| IBIS file p1010_ibis.ibs generated by Viper version: 2010.05.25
[IBIS Ver]   4.2
[Comment Char]   |_char
[File Name]   p1010_ibis.ibs
[File Rev]   E
[Date]   Mon Feb 18 04:38:39 2013
[Source]
[Notes]   Added models for ddr3 Full & Half strength .
|File Rev A : It is generated with the existing lvcmos & ddr models.
|File Rev B : It is updated with insertion of ddr3 Full & Half strength ddr3 models.
|FIle Rev C : It is further updated with the ddr3 /ddr3l input models with ODT Values for full stregth & Half Strength.
|FIle Rev D : Updated Vinl and Vinh value for ddr3 /ddr3l
|FIle Rev E : Expanded Vin data  for ddr3 /ddr3l
|DDR3/DDR3L Input models with ODT for full strength
|v135_in_wb_fs20_term_40_111
|v135_in_wb_fs20_term_45_110
|v135_in_wb_fs20_term_50_101
|v135_in_wb_fs20_term_50_100
|v135_in_wb_fs20_term_100_011
|v135_in_wb_fs20_noterm_000
|v150_in_wb_fs20_term_40_111
|v150_in_wb_fs20_term_45_110
|v150_in_wb_fs20_term_50_101
|v150_in_wb_fs20_term_60_010
|v150_in_wb_fs20_term_150_001
|v150_in_wb_fs20_noterm_000
|DDR3/DDR3L Input models with ODT for default/Half strength
|v135_in_wb_term_40_111
|v135_in_wb_term_45_110
|v135_in_wb_term_50_101
|v135_in_wb_term_50_100
|v135_in_wb_term_100_011
|v135_in_wb_noterm_000
|v150_in_wb_term_40_111
|v150_in_wb_term_45_110
|v150_in_wb_term_50_101
|v150_in_wb_term_60_010
|v150_in_wb_term_150_001
|v150_in_wb_noterm_000
|V135 corresponds to 1.35 volt ddr3l ibis model
|V150 corresponds to 1.50 volt ddr3 ibis model
[Disclaimer] IMPORTANT NOTICE
  This information is provided on an AS IS basis and without warranty.
  IN NO EVENT SHALL Freescale BE LIABLE FOR INCIDENTAL OR CONSEQUENTIAL
  DAMAGES ARISING FROM USE OF THIS INFORMATION. THIS DISCLAIMER OF
  WARRANTY EXTENDS TO THE USER OF THE INFORMATION, AND TO THEIR CUSTOMERS
  OR USERS OF PRODUCTS  AND IS IN LIEU OF ALL WARRANTIES WHETHER EXPRESS,
  IMPLIED, OR STATUTORY, INCLUDING IMPLIED WARRANTIES OF MERCHANTABILITY
  OR FITNESS FOR PARTICULAR PURPOSE.
  Freescale does not represent or warrant that the information furnished
  hereunder is free of infringement of any third party patents,
  copyrights, trade secrets, or other intellectual property rights.
  Freescale does not represent or warrant that the information is free of
  defect, or that it meets any particular standard, requirements or need
  of the user of the infomation or their customers.
  Freescale reserves the right to change the information in this file
  without notice.
[Copyright]   (C) Copyright Freescale 2004 - 2010, All Rights Reserved.
|   P1010
[Component]   P1010
[Manufacturer]   FREESCALE
[Package]
| variable   typ   min   max
R_pkg   0.5638290   0.004778   0.709444
L_pkg   4.99081nH   0.08270nH   8.13625nH
C_pkg   1.95489pF   0.77573pF   61.6917pF
[Pin] signal_name   model_name   R_pin   L_pin   C_pin
A1   VSS   GND   NA   NA   NA
A2   MA4   ddr3_lp   0.669707  7.47435nH 1.33505pF
A3   MA7   ddr3_lp   0.637736  6.2879nH  1.1992pF
A4   MA11   ddr3_lp   0.632318  6.08385nH 1.06391pF
A5   MA6   ddr3_lp   0.616007  5.85776nH 1.13647pF
A6   MA13   ddr3_lp   0.647612  6.15309nH 0.92985pF
A7   MA15   ddr3_lp   0.639758  6.02845nH 0.99263pF
A8   MCS2_B   ddr3_lp   0.588837  6.64056nH 0.93350pF
A9   VSS   GND   NA   NA   NA
A10   S2VDD   POWER   0.0536342 0.77289nH 10.8238pF
A11   SD2_RXE_P   ptrmr100_cm   0.617825  4.91248nH 1.00415pF
A12   S2VDD   POWER   0.0536342 0.77289nH 10.8238pF
A13   SD2_RXA_P   ptrmr100_cm   0.651909  5.19846nH 0.88242pF
A14   X2VDD   POWER   0.0841892 1.09167nH 7.24723pF
A15   VSS   GND   NA   NA   NA
A16   SPI_MOSI   lvcmos   0.625378  6.00035nH 1.0182pF
A17   CAN1_TX   lvcmos   0.611521  5.40587nH 1.08898pF
A18   CAN2_TX   lvcmos   0.638959  6.18092nH 1.00055pF
A19   UART_CTS_B00   lvcmos   0.638349  5.85583nH 0.93401pF
A20   UART_CTS_B01   lvcmos   0.662822  6.52645nH 0.90542pF
A21   IIC1_SDA   lvcmos   0.693375  6.89901nH 1.03172pF
A22   IIC2_SDA   lvcmos   0.690978  6.7034nH  1.2023pF
A23   GPIO02   lvcmos   0.670586  6.92508nH 1.28436pF
B1   MCS0_B   ddr3_lp   0.633996  6.98587nH 1.34917pF
B3   MA3   ddr3_lp   0.673586  6.26512nH 1.29594pF
B4   VSS   GND   NA   NA   NA
B5   MA9   ddr3_lp   0.647296  5.55788nH 1.12941pF
B6   MA2   ddr3_lp   0.628027  5.34605nH 1.05351pF
B7   VSS   GND   NA   NA   NA
B8   MCS3_B   ddr3_lp   0.627363  6.05786nH 0.91183pF
B9   X2VDD   POWER   0.0841892 1.09167nH 7.24723pF
B10   S2VSS   GND   NA   NA   NA
B11   SD2_RXE_N   ptrmr100_cm   0.619546  4.93621nH 1.04449pF
B12   S2VSS   GND   NA   NA   NA
B13   SD2_RXA_N   ptrmr100_cm   0.641883  5.19633nH 0.86855pF
B14   X2VSS   GND   NA   NA   NA
B15   X2VSS   GND   NA   NA   NA
B16   SPI_MISO   lvcmos   0.576792  5.7496nH  1.05876pF
B17   VSS   GND   NA   NA   NA
B18   CAN2_RX   lvcmos   0.561266  4.84225nH 1.13305pF
B19   VSS   GND   NA   NA   NA
B20   IIC1_SCL   lvcmos   0.619918  5.55105nH 1.20145pF
B21   GPIO04   lvcmos   0.667179  6.19423nH 1.30918pF
B22   VSS   GND   NA   NA   NA
B23   GPIO03   lvcmos   0.599915  6.11729nH 1.26323pF
C1   MCKE1   ddr3_lp   0.610929  6.46005nH 1.3986pF
C2   MCS1_B   ddr3_lp   0.566315  6.21152nH 1.28084pF
C3   MA14   ddr3_lp   0.666391  6.00916nH 1.29268pF
C4   MBA0   ddr3_lp   0.601323  5.2337nH  1.2176pF
C5   MBA1   ddr3_lp   0.628619  5.18829nH 1.03111pF
C6   MA8   ddr3_lp   0.595826  5.24786nH 1.32086pF
C7   MA5   ddr3_lp   0.58023   5.04038nH 1.11881pF
C8   MDIC1   ddr3_lp   0.559   4.86888nH 0.90609pF
C9   X2VDD   POWER   0.0841892 1.09167nH 7.24723pF
C10   SD2_TXE_P   ohsdr100   0.656856  4.68821nH 0.88615pF
C11   S2VDD   POWER   0.0536342 0.77289nH 10.8238pF
C12   SD2_REF_CLK   ptrmr100_cm   0.564658  4.23888nH 0.99470pF
C13   X2VDD   POWER   0.0841892 1.09167nH 7.24723pF
C14   SD2_TXA_P   ohsdr100   0.558108  4.46806nH 0.87142pF
C15   S2VDD   POWER   0.0536342 0.77289nH 10.8238pF
C16   SPI_CLK   lvcmos   0.592865  5.07702nH 0.95951pF
C17   OVDD   POWER   0.042658  0.54107nH 23.3177pF
C18   UART_SOUT00   lvcmos   0.603178  5.07125nH 1.04954pF
C19   UART_RTS_B00   lvcmos   0.574586  5.04132nH 0.95538pF
C20   UART_SOUT01   lvcmos   0.642107  5.6184nH  1.07095pF
C21   IIC2_SCL   lvcmos   0.575624  5.12243nH 1.20892pF
C22   OVDD   POWER   0.042658  0.54107nH 23.3177pF
C23   IRQ03   lvcmos   0.591523  6.09858nH 1.23886pF
D1   MA10   ddr3_lp   0.652694  6.26238nH 1.14918pF
D2   VSS   GND   NA   NA   NA
D3   MA0   ddr3_lp   0.584919  5.18099nH 1.12312pF
D4   MBA2   ddr3_lp   0.568256  4.61126nH 1.22577pF
D5   MA12   ddr3_lp   0.597172  4.55009nH 1.2402pF
D6   VSS   GND   NA   NA   NA
D7   MA1   ddr3_lp   0.614011  4.81185nH 1.05428pF
D8   MDIC0   ddr3_lp   0.557983  4.62236nH 1.11328pF
D9   X2VSS   GND   NA   NA   NA
D10   SD2_TXE_N   ohsdr100   0.661854  4.48826nH 0.85457pF
D11   S2VSS   GND   NA   NA   NA
D12   SD2_REF_CLK_B   ptrmr100_cm   0.564493  4.02251nH 1.00229pF
D13   X2VSS   GND   NA   NA   NA
D14   SD2_TXA_N   ohsdr100   0.562706  4.38994nH 0.88457pF
D15   S2VSS   GND   NA   NA   NA
D16   SPI_CS0_B   lvcmos   0.527813  4.60354nH 0.87036pF
D17   CAN1_RX   lvcmos   0.53324   4.36991nH 1.05593pF
D18   UART_SIN00   lvcmos   0.549444  4.60296nH 0.93681pF
D19   UART_RTS_B01   lvcmos   0.581988  4.86482nH 1.12041pF
D20   OVDD   POWER   0.042658  0.54107nH 23.3177pF
D21   IRQ_OUT_B   lvcmos   0.52748   4.74673nH 1.12052pF
D22   GPIO01   lvcmos   0.618068  5.63539nH 1.16022pF
D23   GPIO00   lvcmos   0.574577  5.86541nH 0.97284pF
E1   MODT1   ddr3_lp   0.618133  5.97856nH 1.13831pF
E2   MODT0   ddr3_lp   0.589608  5.34568nH 1.12956pF
E3   MCKE0   ddr3_lp   0.621266  5.21113nH 1.09608pF
E4   VSS   GND   NA   NA   NA
E20   UART_SIN01   lvcmos   0.583707  5.28053nH 1.3149pF
E21   IRQ01   lvcmos   0.539049  4.61628nH 1.16671pF
E22   GPIO05   lvcmos   0.615158  5.9928nH  0.94547pF
E23   HRESET_B   lvcmos   0.607409  6.05555nH 0.91990pF
F1   MRAS_B   ddr3_lp   0.65092   5.87401nH 1.15683pF
F2   MCAS_B   ddr3_lp   0.646409  5.93942nH 1.07527pF
F3   MCK_B   ddr3_lp   0.59967   4.96652nH 1.08589pF
F4   MWE_B   ddr3_lp   0.579535  4.91375nH 1.44213pF
F20   RTC   lvcmos   0.54121   5.18866nH 1.34125pF
F21   READY   lvcmos   0.531341  4.64468nH 1.15887pF
F22   IRQ02   lvcmos   0.54849   5.18259nH 0.96081pF
F23   IRQ00   lvcmos   0.674532  8.13625nH 1.09624pF
G1   MDQ10   ddr3_lp   0.598591  5.87285nH 0.90719pF
G2   VSS   GND   NA   NA   NA
G3   MDQ6   ddr3_lp   0.582092  5.1969nH  1.23341pF
G4   MCK   ddr3_lp   0.547849  4.47303nH 1.10097pF
G7   GVDD   POWER   0.0185408 0.23132nH 61.6917pF
G8   GVDD   POWER   0.0185408 0.23132nH 61.6917pF
G9   GVDD   POWER   0.0185408 0.23132nH 61.6917pF
G10   SD2_IMP_CAL_TX   tx_pzctl   0.586146  5.11116nH 1.01829pF
G11   SD2_PLL_TPA   opdalg_out   0.642874  5.21064nH 1.07289pF
G12   SD2_AVDD   POWER   0.561718  4.85912nH 1.09328pF
G13   SD2_PLL_TPD   pouv_out   0.663651  6.0247nH  1.14914pF
G14   SD2_IMP_CAL_RX   rx_pzctl   0.579436  4.55853nH 1.01843pF
G15   VDD   POWER   0.004778  0.08270nH 54.3076pF
G16   VDD   POWER   0.004778  0.08270nH 54.3076pF
G17   BVDD_VSEL0   lvcmos   0.476143  3.72515nH 1.40013pF
G20   OVDD   POWER   0.042658  0.54107nH 23.3177pF
G21   TCK   lvcmos   0.523466  4.8328nH  0.90469pF
G22   VSS   GND   NA   NA   NA
G23   TDO   lvcmos   0.597779  5.48416nH 1.01916pF
H1   MDQ12   ddr3_lp   0.627741  5.58079nH 0.97414pF
H2   MDQ8   ddr3_lp   0.62387   5.43848nH 0.97839pF
H3   MDQS0   ddr3_lp   0.544829  4.25025nH 1.02585pF
H4   VSS   GND   NA   NA   NA
H7   GVDD   POWER   0.0185408 0.23132nH 61.6917pF
H8   VDD   POWER   0.004778  0.08270nH 54.3076pF
H9   AVDD_CORE   POWER   0.248588  2.75279nH 1.5298pF
H10   VDD   POWER   0.004778  0.08270nH 54.3076pF
H11   VDD   POWER   0.004778  0.08270nH 54.3076pF
H12   SD2_AVSS   POWER   NA   NA   NA
H13   S2VDD   POWER   0.0536342 0.77289nH 10.8238pF
H14   VDD   POWER   0.004778  0.08270nH 54.3076pF
H15   VDD   POWER   0.004778  0.08270nH 54.3076pF
H16   VDD   POWER   0.004778  0.08270nH 54.3076pF
H17   BVDD_VSEL1   lvcmos   0.566016  5.06633nH 1.24902pF
H20   TRST_B   lvcmos   0.556458  4.6237nH  1.05292pF
H21   SCAN_MODE_B   lvcmos   0.550877  4.48222nH 0.93637pF
H22   TDI   lvcmos   0.518741  4.80812nH 0.92720pF
H23   HRESET_REQ_B   lvcmos   0.608453  6.13777nH 0.88758pF
J1   MDQS1   ddr3_lp   0.603453  5.21915nH 0.99317pF
J2   MDQ14   ddr3_lp   0.549859  4.57759nH 0.96075pF
J3   MDQS0_B   ddr3_lp   0.586503  4.49231nH 0.98297pF
J4   MDQ2   ddr3_lp   0.540301  4.47563nH 1.27531pF
J7   MVREF   POWER   0.172675  2.10331nH 1.14195pF
J8   VDD   POWER   0.004778  0.08270nH 54.3076pF
J9   VSS   GND   NA   NA   NA
J10   VSS   GND   NA   NA   NA
J11   VSS   GND   NA   NA   NA
J12   VSS   GND   NA   NA   NA
J13   VSS   GND   NA   NA   NA
J14   VSS   GND   NA   NA   NA
J15   VSS   GND   NA   NA   NA
J16   VDD   POWER   0.004778  0.08270nH 54.3076pF
J17   VDD   POWER   0.004778  0.08270nH 54.3076pF
J20   OVDD   POWER   0.042658  0.54107nH 23.3177pF
J21   USB1_8VDD   POWER   0.145995  2.88747nH 2.6407pF
J22   TMS   lvcmos   0.529573  5.24655nH 0.82968pF
J23   USBVSS   GND   NA   NA   NA
K1   MDQS1_B   ddr3_lp   0.546893  4.81488nH 0.97444pF
K2   VSS   GND   NA   NA   NA
K3   MDQ4   ddr3_lp   0.583367  4.7411nH  0.94803pF
K4   MDQ0   ddr3_lp   0.568442  4.32488nH 1.04202pF
K7   GVDD   POWER   0.0185408 0.23132nH 61.6917pF
K8   VDD   POWER   0.004778  0.08270nH 54.3076pF
K9   VSS   GND   NA   NA   NA
K10   VSS   GND   NA   NA   NA
K11   VSS   GND   NA   NA   NA
K12   VSS   GND   NA   NA   NA
K13   VSS   GND   NA   NA   NA
K14   VSS   GND   NA   NA   NA
K15   VSS   GND   NA   NA   NA
K16   VDD   POWER   0.004778  0.08270nH 54.3076pF
K17   VDD   POWER   0.004778  0.08270nH 54.3076pF
K20   USB3_3VDD   POWER   0.0885715 1.94829nH 2.67041pF
K21   USB1_8VDD   POWER   0.145995  2.88747nH 2.6407pF
K22   USBVSS   GND   NA   NA   NA
K23   UDP   usbphy_utmi   0.637131  4.8277nH  0.85066pF
L1   MDQ9   ddr3_lp   0.551339  5.19313nH 0.83706pF
L2   MDM1   ddr3_lp   0.579481  4.69411nH 0.90271pF
L3   MDQ7   ddr3_lp   0.517179  4.15893nH 1.06703pF
L4   VSS   GND   NA   NA   NA
L7   GVDD   POWER   0.0185408 0.23132nH 61.6917pF
L8   VDD   POWER   0.004778  0.08270nH 54.3076pF
L9   VSS   GND   NA   NA   NA
L10   VSS   GND   NA   NA   NA
L11   VSS   GND   NA   NA   NA
L12   VSS   GND   NA   NA   NA
L13   VSS   GND   NA   NA   NA
L14   VSS   GND   NA   NA   NA
L15   VSS   GND   NA   NA   NA
L16   VDD   POWER   0.004778  0.08270nH 54.3076pF
L17   USB1_0VDD   POWER   0.0763185 0.98405nH 4.57888pF
L20   USB3_3VDD   POWER   0.0885715 1.94829nH 2.67041pF
L21   VBUSCLMP   usbphy_utmi   0.619601  4.57246nH 0.91789pF
L22   USBVSS   GND   NA   NA   NA
L23   UDM   usbphy_utmi   0.636501  4.84494nH 0.95632pF
M1   MDQ15   ddr3_lp   0.572176  5.87759nH 0.94547pF
M2   MDQ11   ddr3_lp   0.591649  5.22724nH 0.77573pF
M3   MDQ1   ddr3_lp   0.569631  4.63143nH 0.95814pF
M4   MDM0   ddr3_lp   0.566079  4.55252nH 1.17114pF
M7   GVDD   POWER   0.0185408 0.23132nH 61.6917pF
M8   VDD   POWER   0.004778  0.08270nH 54.3076pF
M9   VSS   GND   NA   NA   NA
M10   VSS   GND   NA   NA   NA
M11   VSS   GND   NA   NA   NA
M12   VSS   GND   NA   NA   NA
M13   VSS   GND   NA   NA   NA
M14   VSS   GND   NA   NA   NA
M15   VSS   GND   NA   NA   NA
M16   VDD   POWER   0.004778  0.08270nH 54.3076pF
M17   USB1_0VDD   POWER   0.0763185 0.98405nH 4.57888pF
M20   USBPHY_CLK   lvcmos   0.507591  3.98442nH 0.85170pF
M21   USBVSS   GND   NA   NA   NA
M22   IBIAS_REXT   usbphy_utmi   0.627007  4.49729nH 0.83391pF
M23   USBVSS   GND   NA   NA   NA
N1   MDQ13   ddr3_lp   0.539688  4.82707nH 0.93220pF
N2   VSS   GND   NA   NA   NA
N3   MDQ5   ddr3_lp   0.560074  4.49229nH 0.97117pF
N4   MDQ3   ddr3_lp   0.495101  3.70419nH 1.16423pF
N7   GVDD   POWER   0.0185408 0.23132nH 61.6917pF
N8   VDD   POWER   0.004778  0.08270nH 54.3076pF
N9   VSS   GND   NA   NA   NA
N10   VSS   GND   NA   NA   NA
N11   VSS   GND   NA   NA   NA
N12   VSS   GND   NA   NA   NA
N13   VSS   GND   NA   NA   NA
N14   VSS   GND   NA   NA   NA
N15   VSS   GND   NA   NA   NA
N16   VDD   POWER   0.004778  0.08270nH 54.3076pF
N17   AVDD_DDR   POWER   0.219326  1.93282nH 0.88496pF
N20   POVDD2   POWER   0.542753  4.32644nH 0.92698pF
N21   FA_VDD   POWER   0.561498  4.88578nH 0.80055pF
N23   UID   usbphy_utmi   0.646099  5.36988nH 0.82527pF
P1   MDQ26   ddr3_lp   0.596634  5.62472nH 0.84719pF
P2   MDQ30   ddr3_lp   0.51473   4.20885nH 1.00254pF
P3   MDQ22   ddr3_lp   0.516197  4.28499nH 1.03495pF
P4   VSS   GND   NA   NA   NA
P7   GVDD   POWER   0.0185408 0.23132nH 61.6917pF
P8   VDD   POWER   0.004778  0.08270nH 54.3076pF
P9   VSS   GND   NA   NA   NA
P10   VSS   GND   NA   NA   NA
P11   VSS   GND   NA   NA   NA
P12   VSS   GND   NA   NA   NA
P13   VSS   GND   NA   NA   NA
P14   VSS   GND   NA   NA   NA
P15   VSS   GND   NA   NA   NA
P16   VDD   POWER   0.004778  0.08270nH 54.3076pF
P17   AVDD_PLAT   POWER   0.179069  2.26064nH 0.92741pF
P20   VSS   GND   NA   NA   NA
P21   IFC_AD00   lvcmos   0.549024  4.62378nH 0.92908pF
P22   POVDD1   POWER   0.506111  4.44446nH 0.93599pF
P23   SYSCLK   lvcmos   0.529556  4.99071nH 0.93376pF
R1   MDQ28   ddr3_lp   0.548641  5.28194nH 0.83335pF
R2   MDQ24   ddr3_lp   0.581092  5.04501nH 0.97111pF
R3   MDQ18   ddr3_lp   0.498562  3.86987nH 0.94768pF
R4   MDQ16   ddr3_lp   0.559646  4.51877nH 1.20642pF
R7   GVDD   POWER   0.0185408 0.23132nH 61.6917pF
R8   VDD   POWER   0.004778  0.08270nH 54.3076pF
R9   VSS   GND   NA   NA   NA
R10   VSS   GND   NA   NA   NA
R11   VSS   GND   NA   NA   NA
R12   VSS   GND   NA   NA   NA
R13   VSS   GND   NA   NA   NA
R14   VSS   GND   NA   NA   NA
R15   VSS   GND   NA   NA   NA
R16   VDD   POWER   0.004778  0.08270nH 54.3076pF
R17   VDD   POWER   0.004778  0.08270nH 54.3076pF
R20   IFC_AD09   lvcmos   0.53628   4.72182nH 1.05007pF
R21   IFC_AD08   lvcmos   0.5608   4.75575nH 1.10648pF
R22   IFC_AD01   lvcmos   0.526148  4.88108nH 1.05984pF
R23   VSS   GND   NA   NA   NA
T1   MDQS3   ddr3_lp   0.525676  4.60249nH 1.10191pF
T2   VSS   GND   NA   NA   NA
T3   MDQS2   ddr3_lp   0.508487  3.9276nH  1.02701pF
T4   MDQ20   ddr3_lp   0.580586  4.95422nH 1.06341pF
T7   GVDD   POWER   0.0185408 0.23132nH 61.6917pF
T8   VDD   POWER   0.004778  0.08270nH 54.3076pF
T9   VDD   POWER   0.004778  0.08270nH 54.3076pF
T10   VDD   POWER   0.004778  0.08270nH 54.3076pF
T11   X1VDD   POWER   0.0426278 0.54850nH 11.1952pF
T12   SD1_AVSS   POWER   NA   NA   NA
T13   S1VDD   POWER   0.030858  0.41179nH 18.7477pF
T14   VDD   POWER   0.004778  0.08270nH 54.3076pF
T15   VDD   POWER   0.004778  0.08270nH 54.3076pF
T16   VDD   POWER   0.004778  0.08270nH 54.3076pF
T17   BVDD   POWER   0.0563498 0.55906nH 24.8234pF
T20   IFC_AD11   lvcmos   0.556475  4.42435nH 1.13271pF
T21   IFC_AD10   lvcmos   0.561796  4.67054nH 1.05652pF
T22   IFC_AD03   lvcmos   0.576518  5.24186nH 1.04991pF
T23   IFC_AD02   lvcmos   0.554866  5.85041nH 0.94842pF
U1   MDQS3_B   ddr3_lp   0.576591  5.01252nH 1.04675pF
U2   MDQ31   ddr3_lp   0.575304  4.74883nH 1.00082pF
U3   MDQS2_B   ddr3_lp   0.561955  4.34675nH 1.00149pF
U4   VSS   GND   NA   NA   NA
U7   LVDD   POWER   0.0945382 0.90645nH 4.73798pF
U8   LVDD   POWER   0.0945382 0.90645nH 4.73798pF
U9   VDD   POWER   0.004778  0.08270nH 54.3076pF
U10   SD1_IMP_CAL_RX   rx_pzctl   0.623188  4.43113nH 1.09818pF
U11   SD1_PLL_TPD   pouv_out   0.613133  4.74008nH 1.22836pF
U12   SD1_AVDD   POWER   0.665112  4.90282nH 1.31594pF
U13   SD1_PLL_TPA   opdalg_out   0.605487  4.45169nH 1.46565pF
U14   SD1_IMP_CAL_TX   tx_pzctl   0.618011  4.58825nH 1.08525pF
U15   VDD   POWER   0.004778  0.08270nH 54.3076pF
U16   BVDD   POWER   0.0563498 0.55906nH 24.8234pF
U17   BVDD   POWER   0.0563498 0.55906nH 24.8234pF
U20   BVDD   POWER   0.0563498 0.55906nH 24.8234pF
U21   IFC_AD12   lvcmos   0.571067  4.57655nH 1.13147pF
U22   IFC_AD05   lvcmos   0.539649  5.19294nH 1.07278pF
U23   IFC_AD04   lvcmos   0.550187  5.3396nH  1.13308pF
V1   MDM3   ddr3_lp   0.566345  5.58621nH 0.92891pF
V2   MDQ25   ddr3_lp   0.616258  5.46975nH 1.01061pF
V3   MDQ23   ddr3_lp   0.541335  4.57091nH 1.01914pF
V4   MDQ17   ddr3_lp   0.534982  4.27413nH 1.10648pF
V20   IFC_AD14   lvcmos   0.587088  5.51747nH 1.38147pF
V21   IFC_AD13   lvcmos   0.5339   4.74299nH 1.10171pF
V22   IFC_AD07   lvcmos   0.551937  5.25486nH 1.08338pF
V23   IFC_AD06   lvcmos   0.613342  6.34765nH 0.97429pF
W1   MDQ27   ddr3_lp   0.581801  5.88442nH 0.98735pF
W2   VSS   GND   NA   NA   NA
W3   MDM2   ddr3_lp   0.596511  5.07869nH 1.0469pF
W4   MDQ19   ddr3_lp   0.536314  4.39662nH 1.08523pF
W20   IFC_AD15   lvcmos   0.549118  5.79896nH 1.40846pF
W21   IFC_ADDR17   lvcmos   0.553545  5.05151nH 1.15955pF
W22   VSS   GND   NA   NA   NA
W23   IFC_ADDR16   lvcmos   0.590177  6.02005nH 0.97678pF
Y1   MDQ29   ddr3_lp   0.605462  5.74234nH 1.10355pF
Y2   MDQ21   ddr3_lp   0.602782  5.28085nH 1.11815pF
Y3   SENSEVSS   POWER   NA   NA   NA
Y4   VSS   GND   NA   NA   NA
Y5   TSEC1_GTX_CLK125   lvcmos   0.579995  4.90639nH 1.44521pF
Y6   TSEC1_RX_CLK   lvcmos   0.601537  5.43694nH 1.21582pF
Y7   S1VDD   POWER   0.030858  0.41179nH 18.7477pF
Y8   SD1_RXA_P   ptrmr100_cm   0.609394  4.37181nH 0.96637pF
Y9   X1VDD   POWER   0.0426278 0.54850nH 11.1952pF
Y10   SD1_TXB_P   ohsdr100   0.569894  4.15323nH 0.87832pF
Y11   S1VSS   GND   NA   NA   NA
Y12   SD1_REF_CLK_B   ptrmr100_cm   0.589195  3.99843nH 1.01985pF
Y13   S1VDD   POWER   0.030858  0.41179nH 18.7477pF
Y14   SD1_TXE_P   ohsdr100   0.572794  4.08642nH 0.88152pF
Y15   X1VDD   POWER   0.0426278 0.54850nH 11.1952pF
Y16   SD1_RXF_P   ptrmr100_cm   0.607688  4.31003nH 0.98148pF
Y17   S1VSS   GND   NA   NA   NA
Y18   IFC_CLK00   lvcmos   0.624583  5.02031nH 1.08918pF
Y19   IFC_RB_B   lvcmos   0.588781  5.3273nH  1.22473pF
Y20   VSS   GND   NA   NA   NA
Y21   IFC_ADDR21   lvcmos   0.533745  4.63741nH 1.29051pF
Y22   IFC_ADDR19   lvcmos   0.613849  5.49373nH 1.07584pF
Y23   IFC_ADDR18   lvcmos   0.592346  5.67084nH 1.10217pF
AA1   TEMP_ANODE   POWER   0.582631  5.62267nH 1.17374pF
AA2   SENSEVDD   POWER   0.590979  5.0805nH  1.1621pF
AA3   TSEC1_GTX_CLK   lvcmos   0.630901  5.08333nH 1.28258pF
AA4   TSEC1_TXD03   lvcmos   0.641882  5.27418nH 1.17689pF
AA5   TSEC1_TXD02   lvcmos   0.659127  5.83043nH 1.09107pF
AA6   EC_MDC   lvcmos   0.605078  5.57039nH 0.93867pF
AA7   S1VSS   GND   NA   NA   NA
AA8   SD1_RXA_N   ptrmr100_cm   0.607911  4.48097nH 0.98620pF
AA9   X1VSS   GND   NA   NA   NA
AA10  SD1_TXB_N   ohsdr100   0.573348  4.1586nH  0.88594pF
AA11  S1VDD   POWER   0.030858  0.41179nH 18.7477pF
AA12  SD1_REF_CLK   ptrmr100_cm   0.580614  4.17082nH 1.02814pF
AA13  S1VSS   GND   NA   NA   NA
AA14  SD1_TXE_N   ohsdr100   0.579944  4.09679nH 0.88510pF
AA15  X1VSS   GND   NA   NA   NA
AA16  SD1_RXF_N   ptrmr100_cm   0.606592  4.28845nH 0.97199pF
AA17  S1VDD   POWER   0.030858  0.41179nH 18.7477pF
AA18  IFC_PERR_B   lvcmos   0.603674  5.46804nH 1.16772pF
AA19  IFC_BCTL   lvcmos   0.630104  5.08708nH 1.12092pF
AA20  IFC_CLE   lvcmos   0.618497  5.11338nH 1.21022pF
AA21  IFC_CS_B00   lvcmos   0.570828  5.16138nH 1.24161pF
AA22  IFC_ADDR23   lvcmos   0.594176  5.96287nH 1.19899pF
AA23  IFC_ADDR20   lvcmos   0.67697   7.55948nH 1.17245pF
AB1   TEMP_CATHODE   POWER   0.639811  6.35079nH 1.24521pF
AB2   VSS   GND   NA   NA   NA
AB3   TSEC1_RXD02   lvcmos   0.626156  6.03358nH 1.36787pF
AB4   TSEC1_RXD01   lvcmos   0.629991  5.73479nH 1.20087pF
AB5   LVDD   POWER   0.0945382 0.90645nH 4.73798pF
AB6   TSEC1_RX_DV   lvcmos   0.604807  5.74429nH 0.97078pF
AB7   S1VDD   POWER   0.030858  0.41179nH 18.7477pF
AB8   X1VDD   POWER   0.0426278 0.54850nH 11.1952pF
AB9   SD1_TXA_P   ohsdr100   0.680348  5.16315nH 1.04782pF
AB10  S1VDD   POWER   0.030858  0.41179nH 18.7477pF
AB11  SD1_RXB_P   ptrmr100_cm   0.670078  4.60822nH 0.98997pF
AB12  S1VDD   POWER   0.030858  0.41179nH 18.7477pF
AB13  SD1_RXE_P   ptrmr100_cm   0.663338  4.90241nH 0.97822pF
AB14  S1VDD   POWER   0.030858  0.41179nH 18.7477pF
AB15  SD1_TXF_P   ohsdr100   0.678943  5.05252nH 1.00418pF
AB16  X1VDD   POWER   0.0426278 0.54850nH 11.1952pF
AB17  S1VSS   GND   NA   NA   NA
AB18  IFC_PAR01   lvcmos   0.645234  5.68541nH 1.01064pF
AB19  BVDD   POWER   0.0563498 0.55906nH 24.8234pF
AB20  IFC_OE_B   lvcmos   0.619543  5.82433nH 1.12716pF
AB21  IFC_CS_B01   lvcmos   0.647022  6.27384nH 1.22691pF
AB22  VSS   GND   NA   NA   NA
AB23  IFC_ADDR22   lvcmos   0.655186  6.6605nH  1.20673pF
AC1   TSEC1_TXD01   lvcmos   0.640529  6.43105nH 1.26827pF
AC2   EC_MDIO   lvcmos   0.682069  6.46251nH 1.22748pF
AC3   TSEC1_RXD03   lvcmos   0.709444  7.1316nH  1.08878pF
AC4   TSEC1_RXD00   lvcmos   0.696181  6.83227nH 0.84602pF
AC5   TSEC1_TXD00   lvcmos   0.682234  7.14506nH 1.04788pF
AC6   TSEC1_TX_EN   lvcmos   0.674474  7.34247nH 1.0275pF
AC7   VSS   GND   NA   NA   NA
AC8   X1VSS   GND   NA   NA   NA
AC9   SD1_TXA_N   ohsdr100   0.677065  5.09706nH 1.02841pF
AC10  S1VSS   GND   NA   NA   NA
AC11  SD1_RXB_N   ptrmr100_cm   0.670595  4.73981nH 0.98119pF
AC12  S1VSS   GND   NA   NA   NA
AC13  SD1_RXE_N   ptrmr100_cm   0.664308  5.03691nH 1.00475pF
AC14  S1VSS   GND   NA   NA   NA
AC15  SD1_TXF_N   ohsdr100   0.683267  4.9842nH  0.99502pF
AC16  X1VSS   GND   NA   NA   NA
AC17  VSS   GND   NA   NA   NA
AC18  IFC_CLK01   lvcmos   0.611546  6.28529nH 0.99856pF
AC19  IFC_PAR00   lvcmos   0.617558  5.77543nH 1.17364pF
AC20  IFC_WP_B   lvcmos   0.678552  6.66695nH 0.97154pF
AC21  IFC_WE_B   lvcmos   0.627871  6.33206nH 1.21144pF
AC22  IFC_AVD   lvcmos   0.630515  6.24539nH 1.22264pF
AC23  IFC_ADDR24   lvcmos   0.588367  6.65852nH 1.25291pF
[Pin Mapping]   pulldown_ref   pullup_ref
A1   VSS   NC
A2   NC   GVDD
A3   NC   GVDD
A4   NC   GVDD
A5   NC   GVDD
A6   NC   GVDD
A7   NC   GVDD
A8   NC   GVDD
A9   VSS   NC
A10   NC   S2VDD
A11   NC   NC
A12   NC   S2VDD
A13   NC   NC
A14   NC   X2VDD
A15   VSS   NC
A16   NC   OVDD
A17   NC   OVDD
A18   NC   OVDD
A19   NC   OVDD
A20   NC   OVDD
A21   NC   OVDD
A22   NC   OVDD
A23   NC   OVDD
B1   NC   GVDD
B3   NC   GVDD
B4   VSS   NC
B5   NC   GVDD
B6   NC   GVDD
B7   VSS   NC
B8   NC   GVDD
B9   NC   X2VDD
B10   S2VSS   NC
B11   NC   NC
B12   S2VSS   NC
B13   NC   NC
B14   X2VSS   NC
B15   X2VSS   NC
B16   NC   OVDD
B17   VSS   NC
B18   NC   OVDD
B19   VSS   NC
B20   NC   OVDD
B21   NC   OVDD
B22   VSS   NC
B23   NC   OVDD
C1   NC   GVDD
C2   NC   GVDD
C3   NC   GVDD
C4   NC   GVDD
C5   NC   GVDD
C6   NC   GVDD
C7   NC   GVDD
C8   NC   GVDD
C9   NC   X2VDD
C10   NC   NC
C11   NC   S2VDD
C12   NC   NC
C13   NC   X2VDD
C14   NC   NC
C15   NC   S2VDD
C16   NC   OVDD
C17   NC   OVDD
C18   NC   OVDD
C19   NC   OVDD
C20   NC   OVDD
C21   NC   OVDD
C22   NC   OVDD
C23   NC   OVDD
D1   NC   GVDD
D2   VSS   NC
D3   NC   GVDD
D4   NC   GVDD
D5   NC   GVDD
D6   VSS   NC
D7   NC   GVDD
D8   NC   GVDD
D9   X2VSS   NC
D10   NC   NC
D11   S2VSS   NC
D12   NC   NC
D13   X2VSS   NC
D14   NC   NC
D15   S2VSS   NC
D16   NC   OVDD
D17   NC   OVDD
D18   NC   OVDD
D19   NC   OVDD
D20   NC   OVDD
D21   NC   OVDD
D22   NC   OVDD
D23   NC   OVDD
E1   NC   GVDD
E2   NC   GVDD
E3   NC   GVDD
E4   VSS   NC
E20   NC   OVDD
E21   NC   OVDD
E22   NC   OVDD
E23   NC   OVDD
F1   NC   GVDD
F2   NC   GVDD
F3   NC   GVDD
F4   NC   GVDD
F20   NC   OVDD
F21   NC   OVDD
F22   NC   OVDD
F23   NC   OVDD
G1   NC   GVDD
G2   VSS   NC
G3   NC   GVDD
G4   NC   GVDD
G7   NC   GVDD
G8   NC   GVDD
G9   NC   GVDD
G10   NC   NC
G11   NC   NC
G12   NC   SD2_AVDD
G13   NC   NC
G14   NC   NC
G15   NC   VDD
G16   NC   VDD
G17   NC   OVDD
G20   NC   OVDD
G21   NC   OVDD
G22   VSS   NC
G23   NC   OVDD
H1   NC   GVDD
H2   NC   GVDD
H3   NC   GVDD
H4   VSS   NC
H7   NC   GVDD
H8   NC   VDD
H9   NC   GVDD
H10   NC   VDD
H11   NC   VDD
H12   NC   SD2_AVSS
H13   NC   S2VDD
H14   NC   VDD
H15   NC   VDD
H16   NC   VDD
H17   NC   OVDD
H20   NC   OVDD
H21   NC   OVDD
H22   NC   OVDD
H23   NC   OVDD
J1   NC   GVDD
J2   NC   GVDD
J3   NC   GVDD
J4   NC   GVDD
J7   NC   GVDD
J8   NC   VDD
J9   VSS   NC
J10   VSS   NC
J11   VSS   NC
J12   VSS   NC
J13   VSS   NC
J14   VSS   NC
J15   VSS   NC
J16   NC   VDD
J17   NC   VDD
J20   NC   OVDD
J21   NC   USB1_8VDD
J22   NC   OVDD
J23   USBVSS   NC
K1   NC   GVDD
K2   VSS   NC
K3   NC   GVDD
K4   NC   GVDD
K7   NC   GVDD
K8   NC   VDD
K9   VSS   NC
K10   VSS   NC
K11   VSS   NC
K12   VSS   NC
K13   VSS   NC
K14   VSS   NC
K15   VSS   NC
K16   NC   VDD
K17   NC   VDD
K20   NC   USB3_3VDD
K21   NC   USB1_8VDD
K22   USBVSS   NC
K23   NC   NC
L1   NC   GVDD
L2   NC   GVDD
L3   NC   GVDD
L4   VSS   NC
L7   NC   GVDD
L8   NC   VDD
L9   VSS   NC
L10   VSS   NC
L11   VSS   NC
L12   VSS   NC
L13   VSS   NC
L14   VSS   NC
L15   VSS   NC
L16   NC   VDD
L17   NC   USB1_0VDD
L20   NC   USB3_3VDD
L21   NC   NC
L22   USBVSS   NC
L23   NC   NC
M1   NC   GVDD
M2   NC   GVDD
M3   NC   GVDD
M4   NC   GVDD
M7   NC   GVDD
M8   NC   VDD
M9   VSS   NC
M10   VSS   NC
M11   VSS   NC
M12   VSS   NC
M13   VSS   NC
M14   VSS   NC
M15   VSS   NC
M16   NC   VDD
M17   NC   USB1_0VDD
M20   NC   OVDD
M21   USBVSS   NC
M22   NC   NC
M23   USBVSS   NC
N1   NC   GVDD
N2   VSS   NC
N3   NC   GVDD
N4   NC   GVDD
N7   NC   GVDD
N8   NC   VDD
N9   VSS   NC
N10   VSS   NC
N11   VSS   NC
N12   VSS   NC
N13   VSS   NC
N14   VSS   NC
N15   VSS   NC
N16   NC   VDD
N17   NC   OVDD
N20   NC   OVDD
N21   NC   OVDD
N23   NC   NC
P1   NC   GVDD
P2   NC   GVDD
P3   NC   GVDD
P4   VSS   NC
P7   NC   GVDD
P8   NC   VDD
P9   VSS   NC
P10   VSS   NC
P11   VSS   NC
P12   VSS   NC
P13   VSS   NC
P14   VSS   NC
P15   VSS   NC
P16   NC   VDD
P17   NC   OVDD
P20   VSS   NC
P21   NC   BVDD
P22   NC   OVDD
P23   NC   OVDD
R1   NC   GVDD
R2   NC   GVDD
R3   NC   GVDD
R4   NC   GVDD
R7   NC   GVDD
R8   NC   VDD
R9   VSS   NC
R10   VSS   NC
R11   VSS   NC
R12   VSS   NC
R13   VSS   NC
R14   VSS   NC
R15   VSS   NC
R16   NC   VDD
R17   NC   VDD
R20   NC   BVDD
R21   NC   BVDD
R22   NC   BVDD
R23   VSS   NC
T1   NC   GVDD
T2   VSS   NC
T3   NC   GVDD
T4   NC   GVDD
T7   NC   GVDD
T8   NC   VDD
T9   NC   VDD
T10   NC   VDD
T11   NC   X1VDD
T12   NC   SD1_AVSS
T13   NC   S1VDD
T14   NC   VDD
T15   NC   VDD
T16   NC   VDD
T17   NC   BVDD
T20   NC   BVDD
T21   NC   BVDD
T22   NC   BVDD
T23   NC   BVDD
U1   NC   GVDD
U2   NC   GVDD
U3   NC   GVDD
U4   VSS   NC
U7   NC   LVDD
U8   NC   LVDD
U9   NC   VDD
U10   NC   NC
U11   NC   NC
U12   NC   SD1_AVDD
U13   NC   NC
U14   NC   NC
U15   NC   VDD
U16   NC   BVDD
U17   NC   BVDD
U20   NC   BVDD
U21   NC   BVDD
U22   NC   BVDD
U23   NC   BVDD
V1   NC   GVDD
V2   NC   GVDD
V3   NC   GVDD
V4   NC   GVDD
V20   NC   BVDD
V21   NC   BVDD
V22   NC   BVDD
V23   NC   BVDD
W1   NC   GVDD
W2   VSS   NC
W3   NC   GVDD
W4   NC   GVDD
W20   NC   BVDD
W21   NC   BVDD
W22   VSS   NC
W23   NC   BVDD
Y1   NC   GVDD
Y2   NC   GVDD
Y3   NC   LVDD
Y4   VSS   NC
Y5   NC   LVDD
Y6   NC   LVDD
Y7   NC   S1VDD
Y8   NC   NC
Y9   NC   X1VDD
Y10   NC   NC
Y11   S1VSS   NC
Y12   NC   NC
Y13   NC   S1VDD
Y14   NC   NC
Y15   NC   X1VDD
Y16   NC   NC
Y17   S1VSS   NC
Y18   NC   BVDD
Y19   NC   BVDD
Y20   VSS   NC
Y21   NC   BVDD
Y22   NC   BVDD
Y23   NC   BVDD
AA1   NC   LVDD
AA2   NC   LVDD
AA3   NC   LVDD
AA4   NC   LVDD
AA5   NC   LVDD
AA6   NC   LVDD
AA7   S1VSS   NC
AA8   NC   NC
AA9   X1VSS   NC
AA10   NC   NC
AA11   NC   S1VDD
AA12   NC   NC
AA13   S1VSS   NC
AA14   NC   NC
AA15   X1VSS   NC
AA16   NC   NC
AA17   NC   S1VDD
AA18   NC   BVDD
AA19   NC   BVDD
AA20   NC   BVDD
AA21   NC   BVDD
AA22   NC   BVDD
AA23   NC   BVDD
AB1   NC   LVDD
AB2   VSS   NC
AB3   NC   LVDD
AB4   NC   LVDD
AB5   NC   LVDD
AB6   NC   LVDD
AB7   NC   S1VDD
AB8   NC   X1VDD
AB9   NC   NC
AB10   NC   S1VDD
AB11   NC   NC
AB12   NC   S1VDD
AB13   NC   NC
AB14   NC   S1VDD
AB15   NC   NC
AB16   NC   X1VDD
AB17   S1VSS   NC
AB18   NC   BVDD
AB19   NC   BVDD
AB20   NC   BVDD
AB21   NC   BVDD
AB22   VSS   NC
AB23   NC   BVDD
AC1   NC   LVDD
AC2   NC   LVDD
AC3   NC   LVDD
AC4   NC   LVDD
AC5   NC   LVDD
AC6   NC   LVDD
AC7   VSS   NC
AC8   X1VSS   NC
AC9   NC   NC
AC10   S1VSS   NC
AC11   NC   NC
AC12   S1VSS   NC
AC13   NC   NC
AC14   S1VSS   NC
AC15   NC   NC
AC16   X1VSS   NC
AC17   VSS   NC
AC18   NC   BVDD
AC19   NC   BVDD
AC20   NC   BVDD
AC21   NC   BVDD
AC22   NC   BVDD
AC23   NC   BVDD
[Diff Pin]  inv_pin  vdiff  tdelay_typ tdelay_min tdelay_max
G4   F3   NA   NA   NA   NA
H3   J3   NA   NA   NA   NA
J1   K1   NA   NA   NA   NA
T3   U3   NA   NA   NA   NA
T1   U1   NA   NA   NA   NA
Y8   AA8   NA   NA   NA   NA
AB11   AC11   NA   NA   NA   NA
AB13   AC13   NA   NA   NA   NA
Y16   AA16   NA   NA   NA   NA
AB9   AC9   NA   NA   NA   NA
Y10   AA10   NA   NA   NA   NA
Y14   AA14   NA   NA   NA   NA
AB15   AC15   NA   NA   NA   NA
A13   B13   NA   NA   NA   NA
A11   B11   NA   NA   NA   NA
C14   D14   NA   NA   NA   NA
C10   D10   NA   NA   NA   NA
|*   Model Selector   *
[Model Selector] usbphy_utmi
usb_FS   USB IO for FS_USB
usb_HS   USB IO for HS_USB
[Model Selector] ddr3_lp
v135_out_wb_term_40_111   DDR1.35 Buffer
v135_out_wb_term_45_110   DDR1.35 Buffer
v135_out_wb_term_50_101   DDR1.35 Buffer
v135_out_wb_term_50_100   DDR1.35 Buffer
v135_out_wb_term_100_011   DDR1.35 Buffer
v135_out_wb_noterm_000   DDR1.35 Buffer
v150_out_wb_term_40_111   DDR1.5 Buffer
v150_out_wb_term_45_110   DDR1.5 Buffer
v150_out_wb_term_50_101   DDR1.5 Buffer
v150_out_wb_term_60_010   DDR1.5 Buffer
v150_out_wb_term_150_001   DDR1.5 Buffer
v150_out_wb_noterm_000   DDR1.5 Buffer
v135_wb_term_40_111   DDR1.35 Receiver
v135_wb_term_45_110   DDR1.35 Receiver
v135_wb_term_50_101   DDR1.35 Receiver
v135_wb_term_50_100   DDR1.35 Receiver
v135_wb_term_100_011   DDR1.35 Receiver
v135_wb_noterm_000   DDR1.35 Receiver
v150_wb_term_40_111   DDR1.5 Receiver
v150_wb_term_45_110   DDR1.5 Receiver
v150_wb_term_50_101   DDR1.5 Receiver
v150_wb_term_60_010   DDR1.5 Receiver
v150_wb_term_150_001   DDR1.5 Receiver
v150_wb_noterm_000   DDR1.5 Receiver
ddr3_drvr_17   DDR1.5 Full Strength
ddr3_drvr_40   DDR1.5 Half Strength
v135_in_wb_fs20_term_40_111   DDR1.35 Full Strength 40 ohm ODT
v135_in_wb_fs20_term_45_110   DDR1.35 Full Strength 45 ohm ODT
v135_in_wb_fs20_term_50_101   DDR1.35 Full Strength 50 ohm ODT
v135_in_wb_fs20_term_50_100   DDR1.35 Full Strength 50 ohm ODT
v135_in_wb_fs20_term_100_011   DDR1.35 Full Strength 100 ohm ODT
v135_in_wb_fs20_noterm_000   DDR1.35 Full Strength no ODT
v150_in_wb_fs20_term_40_111   DDR1.5 Full Strength 40 ohm ODT
v150_in_wb_fs20_term_45_110   DDR1.5 Full Strength 45 ohm ODT
v150_in_wb_fs20_term_50_101   DDR1.5 Full Strength 50 ohm ODT
v150_in_wb_fs20_term_60_010   DDR1.5 Full Strength 60 ohm ODT
v150_in_wb_fs20_term_150_001   DDR1.5 Full Strength 150 ohm ODT
v150_in_wb_fs20_noterm_000   DDR1.5 Full Strength no ODT
v135_in_wb_term_40_111   DDR1.35 Half Strength 40 ohm ODT
v135_in_wb_term_45_110   DDR1.35 Half Strength 45 ohm ODT
v135_in_wb_term_50_101   DDR1.35 Half Strength 50 ohm ODT
v135_in_wb_term_50_100   DDR1.35 Half Strength 50 ohm ODT
v135_in_wb_term_100_011   DDR1.35 Half Strength 100 ohm ODT
v135_in_wb_noterm_000   DDR1.35 Half Strength no ODT
v150_in_wb_term_40_111   DDR1.5 Half Strength 40 ohm ODT
v150_in_wb_term_45_110   DDR1.5 Half Strength 45 ohm ODT
v150_in_wb_term_50_101   DDR1.5 Half Strength 50 ohm ODT
v150_in_wb_term_60_010   DDR1.5 Half Strength 60 ohm ODT
v150_in_wb_term_150_001   DDR1.5 Half Strength 150 ohm ODT
v150_in_wb_noterm_000   DDR1.5 Half Strength no ODT
v150_out_wb_term_150_001_with_pg   DDR1.5 Buffer, with Power and Ground Clamp data added
v150_wb_term_150_001_with_pg   DDR1.5 Receiver, with Power and Ground Clamp data added
[Model Selector] lvcmos
v330_out_od_wb   LVCMOS3.3V Driver(open_drain)
v250_out_od_wb   LVCMOS2.5V Driver(open_drain)
v180_out_od_wb   LVCMOS1.8V Driver(open_drain)
v330_io_od_wb   LVCMOS3.3VIO(open_drain)
v250_io_od_wb   LVCMOS2.5VIO(open_drain)
v180_io_od_wb   LVCMOS1.8VIO(open_drain)
v330_in_wb   LVCMOS3.3V Receiver
v250_in_wb   LVCMOS2.5V Receiver
v180_in_wb   LVCMOS1.8V Receiver
v330_out_wb   LVCMOS3.3V Driver
v250_out_wb   LVCMOS2.5V Driver
v180_out_wb   LVCMOS1.8V Driver
v180_wb   LVCMOS1.8VIO
v250_wb   LVCMOS2.5VIO
v330_wb   LVCMOS3.3VIO
[Model Selector] ohsdr100
sd45_ohsdr100_x_004p   PCI Express:  level 1.5
sd45_ohsdr100_x_006p   PCI Express:  level 2.0
sd45_ohsdr100_x_403   SGMII: level 1.5
sd45_ohsdr100_x_404   SGMII: level 2.0
sd45_ohsdr100_x_502   SATA2: level 1.5
sd45_ohsdr100_x_503   SATA2: level 2.0
sd45_ohsdr100_x_602   SATA1: level 1.5
sd45_ohsdr100_x_603   SATA1: level 2.0
| Models and submodels in the file (94): opdalg_out (Output), pouv_out (3-state), ptrmr100_cm (Input), rx_pzctl (Input), sd45_ohsdr100_x_00 (3-state), sd45_ohsdr100_x_004p (3-state), sd45_ohsdr100_x_006p (3-state), sd45_ohsdr100_x_04 (3-state), sd45_ohsdr100_x_06 (3-state), sd45_ohsdr100_x_40 (3-state), sd45_ohsdr100_x_403 (3-state), sd45_ohsdr100_x_404 (3-state), sd45_ohsdr100_x_43 (3-state), sd45_ohsdr100_x_44 (3-state), tx_pzctl (Input), usb_FS (I/O), usb_HS (I/O), v135_out_wb_noterm_000 (Output), v135_out_wb_term_100_011 (Output), v135_out_wb_term_40_111 (Output), v135_out_wb_term_45_110 (Output), v135_out_wb_term_50_100 (Output), v135_out_wb_term_50_101 (Output), v135_wb_noterm_000 (I/O), v135_wb_term_100_011 (I/O), v135_wb_term_40_111 (I/O), v135_wb_term_45_110 (I/O), v135_wb_term_50_100 (I/O), v135_wb_term_50_101 (I/O), v150_out_wb_noterm_000 (Output), v150_out_wb_term_150_001 (Output), v150_out_wb_term_40_111 (Output), v150_out_wb_term_45_110 (Output), v150_out_wb_term_50_101 (Output), v150_out_wb_term_60_010 (Output), v150_wb_noterm_000 (I/O), v150_wb_term_150_001 (I/O), v150_wb_term_40_111 (I/O), v150_wb_term_45_110 (I/O), v150_wb_term_50_101 (I/O), v150_wb_term_60_010 (I/O), v180_in_wb (Input), v180_io_od_wb (I/O_open_drain), v180_out_od_wb (Open_drain), v180_out_wb (Output), v180_wb (I/O), v250_in_wb (Input), v250_io_od_wb (I/O_open_drain), v250_out_od_wb (Open_drain), v250_out_wb (Output), v250_wb (I/O), v330_in_wb (Input), v330_io_od_wb (I/O_open_drain), v330_out_od_wb (Open_drain), v330_out_wb (Output), v330_wb (I/O), ddr3_drvr_17 (I/O), ddr3_drvr_40 (I/O), sd45_ohsdr100_x_50 (3-state), sd45_ohsdr100_x_502 (3-state), sd45_ohsdr100_x_503 (3-state), sd45_ohsdr100_x_52 (3-state), sd45_ohsdr100_x_53 (3-state), sd45_ohsdr100_x_60 (3-state), sd45_ohsdr100_x_602 (3-state), sd45_ohsdr100_x_603 (3-state), sd45_ohsdr100_x_62 (3-state), sd45_ohsdr100_x_63 (3-state), v150_in_wb_noterm_000 (Input), v150_in_wb_term_150_001 (Input), v150_in_wb_term_60_010 (Input), v150_in_wb_term_50_101 (Input), v150_in_wb_term_45_110 (Input), v150_in_wb_term_40_111 (Input), v135_in_wb_noterm_000 (Input), v135_in_wb_term_100_011 (Input), v135_in_wb_term_50_100 (Input), v135_in_wb_term_50_101 (Input), v135_in_wb_term_45_110 (Input), v135_in_wb_term_40_111 (Input)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
